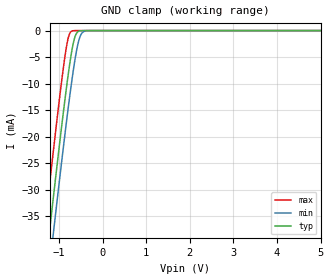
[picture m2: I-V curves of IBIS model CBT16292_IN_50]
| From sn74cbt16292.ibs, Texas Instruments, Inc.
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[Model]   CBT16292_IN_50
Model_type  Input
Vinl = 0.8
Vinh = 2.0
| variable   typ   min   max
C_comp   1.64pF   1.06pF   4.61pF
[Temperature Range]   40   100   -40
| Ambient temperature   25   85   -40
[Voltage range]   5   4.5   5.5
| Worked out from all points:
|   GND clamp passes 1 mA (typ) near -0.63 V on its own axis
[GND Clamp]
| CBT16292_IN_50
|   Voltage   I(typ)   I(min)   I(max)
-5V       -327.3mA   -333.4mA   -319.5mA
-1.365V   -48.74mA   -55.5mA    -40.02mA
-1.325V   -45.78mA   -52.55mA   -37.05mA
-1.215V   -37.7mA    -44.48mA   -28.94mA
-1.125V   -31.16mA   -37.95mA   -22.41mA
-850mV    -12.12mA   -18.65mA   -4.156mA
-780mV    -7.787mA   -14.05mA   -1.143mA
-710mV    -4.013mA   -9.713mA   -111.7uA
-625mV    -978.1uA   -5.059mA   -3.551uA
-540mV    -103.1uA   -1.713mA   -104.2nA
-380mV    -774.4nA   -49uA      -140.7pA
5V        35.05pA    2.725nA    24.17pA
